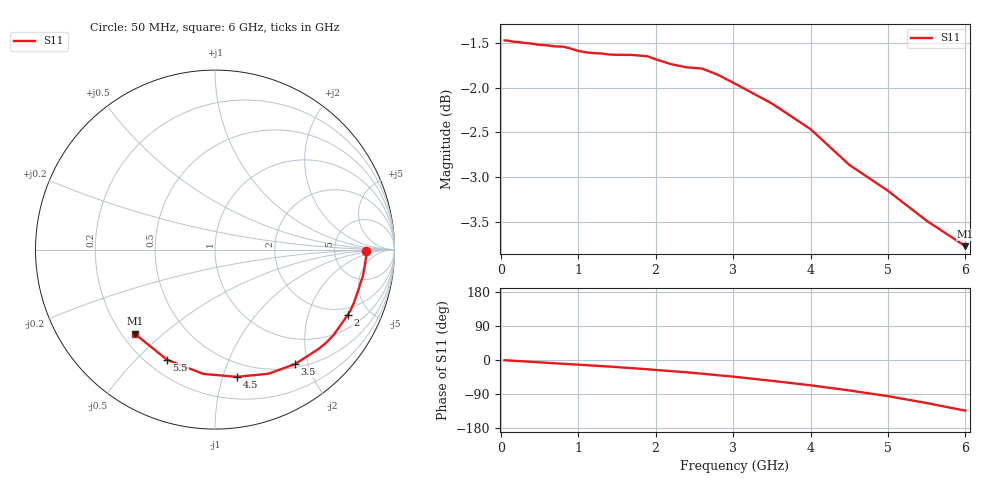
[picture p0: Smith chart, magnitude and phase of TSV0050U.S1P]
! SIEMENS Small Signal Semiconductors
! BAT14-03W
! Si Schottky Diode in SOD323
! IF = 0.05 mA
! S-Parameters:  November  1995
# GHz  S  MA  R  50
!  f  S11
! GHz  MAG  ANG
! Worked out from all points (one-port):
!   34 points, 50 MHz to 6 GHz, reference 50 ohm
!   lowest |S11| = -3.8 dB at 6 GHz (marker M1), VSWR 4.68, Z = 12.5 - j20.2 ohm
!   |S11| at or under -10 dB: nowhere
!   S11 on the Smith chart (normalised r, x): 50 MHz: 12, -1; 2 GHz: 1.59, -3.62; 3.5 GHz: 0.55, -1.79; 4.5 GHz: 0.38, -1.11; 5.5 GHz: 0.28, -0.62; 6 GHz: 0.25, -0.40
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0.05  0.844 -0.7
0.1  0.8438 -1.2
0.15  0.8428 -1.9
0.3  0.8414 -3.7
0.4  0.8405 -5.0
0.6  0.8387 -7.4
0.7  0.8375 -8.7
0.8  0.8374 -9.8
1.1  0.8312 -13.6
1.2  0.8303 -14.8
1.3  0.83 -16.1
1.4  0.8288 -17.3
1.6  0.8285 -20.2
1.7  0.8284 -21.5
1.8  0.8277 -23.1
1.9  0.8269 -24.5
2  0.8238 -26.3
2.2  0.8186 -29.3
2.4  0.8153 -32.5
2.6  0.814 -36.1
2.8  0.8077 -40.1
3  0.7994 -43.8
3.5  0.7783 -55.0
4  0.753 -66.7
4.5  0.7193 -80.3
5  0.6956 -95.4
5.5  0.6693 -113.6
6  0.6478 -133.7
